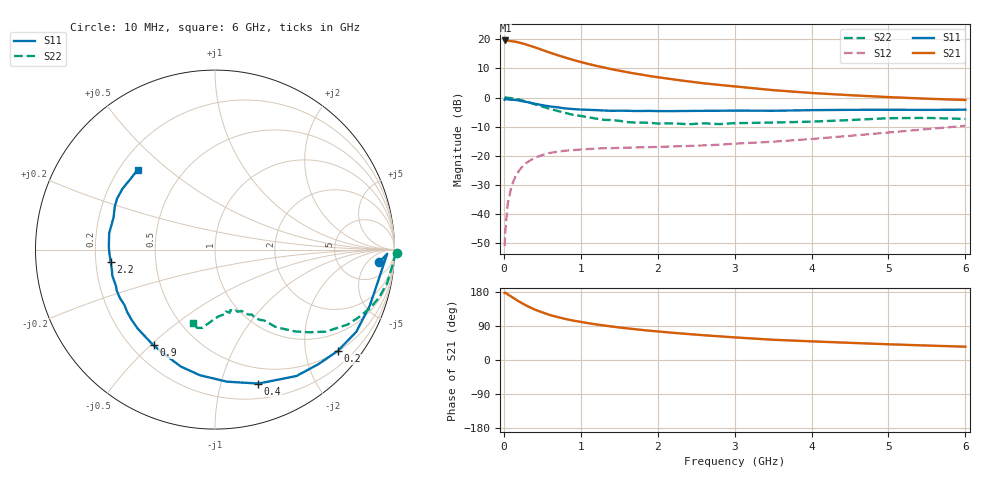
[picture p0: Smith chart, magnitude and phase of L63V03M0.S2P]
!  INFINEON TECHNOLOGIES Small Signal Semiconductors
! BFR380L3 , Si-NPN RF-Transistor in TSLP-3-1
!  Vce=3 V,  Ic=3 mA
! Common Emitter S-Parameters:  07. March 2005
#  GHz  S  MA  R  50
! f  S11  S21  S12  S22
! GHz  Mag  Ang  Mag  Ang  Mag  Ang  Mag  Ang
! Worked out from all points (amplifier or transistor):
!   36 points, 10 MHz to 6 GHz, reference 50 ohm
!   highest |S21| = 19.6 dB at 20 MHz (marker M1)
!   |S21| within 3 dB of that: start of sweep to 472.6 MHz
!   unconditionally stable (mu >= 1): 2.648 GHz to 4.658 GHz
!   at 250 MHz: K = 0.12, MSG = 21.0 dB, |S12| = -23.5 dB
!   at 1.4 GHz: K = 0.64, MSG = 13.6 dB, |S12| = -17.4 dB
!   at 6 GHz: K = 0.91, MSG = 4.4 dB, |S12| = -9.7 dB
!   S11 on the Smith chart (normalised r, x): 10 MHz: 13, -12; 200 MHz: 0.51, -2.69; 400 MHz: 0.34, -1.32; 900 MHz: 0.29, -0.51; 2.2 GHz: 0.26, -0.05; 6 GHz: 0.27, +0.40
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0.01  0.9179 -4.4  9.51 177.0  0.0028 81.1  1.015 -1.1
0.02  0.9597 -1.4  9.569 177.6  0.0052 85.7  1.002 -2.4
0.05  0.9268 -10.3  9.461 173.3  0.0148 86.2  0.9908 -5.5
0.1  0.9172 -19.9  9.297 166.9  0.0302 80.3  0.9769 -11.0
0.15  0.9108 -30.2  9.116 160.4  0.0436 74.4  0.9523 -16.4
0.2  0.887 -39.6  8.805 154.0  0.0561 70.2  0.9224 -20.8
0.3  0.8379 -57.2  8.066 142.8  0.0767 60.7  0.8483 -29.5
0.4  0.7843 -72.1  7.322 133.3  0.0923 53.7  0.7685 -36.5
0.5  0.7387 -84.9  6.578 125.7  0.103 48.9  0.699 -41.2
0.6  0.7048 -96.9  5.906 118.6  0.112 44.2  0.6398 -45.5
0.7  0.679 -106.2  5.339 113.3  0.1174 41.7  0.5887 -48.8
0.8  0.6502 -114.7  4.859 108.3  0.1225 39.2  0.5441 -52.1
0.9  0.634 -122.7  4.434 104.1  0.1251 37.4  0.5045 -53.9
1.1  0.6157 -134.3  3.777 97.0  0.1306 35.7  0.4604 -57.9
1.5  0.5945 -153.0  2.9 85.8  0.1368 35.2  0.3988 -64.0
1.9  0.5899 -165.9  2.338 77.2  0.1407 37.0  0.3685 -70.0
2.2  0.5853 -173.3  2.055 71.7  0.1448 39.5  0.3607 -72.1
2.6  0.5917 178.5  1.757 65.3  0.1507 43.4  0.3612 -77.0
3.5  0.5929 162.4  1.341 53.4  0.1744 52.0  0.372 -86.8
4.5  0.6151 152.4  1.098 45.3  0.2202 60.6  0.4106 -94.8
5.5  0.6137 140.9  0.955 38.2  0.2868 63.7  0.4472 -102.8
6  0.619 134.2  0.908 35.1  0.3269 63.3  0.4298 -106.8
